FUNCTION "FC_GRP_83" : VOID
TITLE =GROUP =83
{ S7_language := '9(1) Angielski (Stany Zjednoczone)  11.01.2022  09:45:15' }
VERSION : 0.1


VAR_TEMP
  CL : "UDT_CABINET";	//CABINET LOCAL
  CR : "UDT_CABINET";	//CABINET REMOTE
  RelError : BOOL ;	//ERROR RELEASE
  RelErrorCL : BOOL ;	//ERROR RELEASE FROM CABINET LOCAL
  RelErrorCR : BOOL ;	//ERROR RELEASE FROM CABINET REMOTE
  RelControl : BOOL ;	//CONTROL RELEASE
  RelControlCL : BOOL ;	//CONTROL RELEASE FROM CABINET LOCAL
  RelControlCR : BOOL ;	//CONTROL RELEASE FROM CABINET REMOTE
  ErrorConfirm : BOOL ;	//ERROR CONFIRM
  AutoOn : BOOL ;	//AUTOMATIC ON
  AutoOff : BOOL ;	//AUTOMATIC OFF
  LAMP_ON : BOOL ;
END_VAR
BEGIN
NETWORK
TITLE =GLOBAL SIGNALS
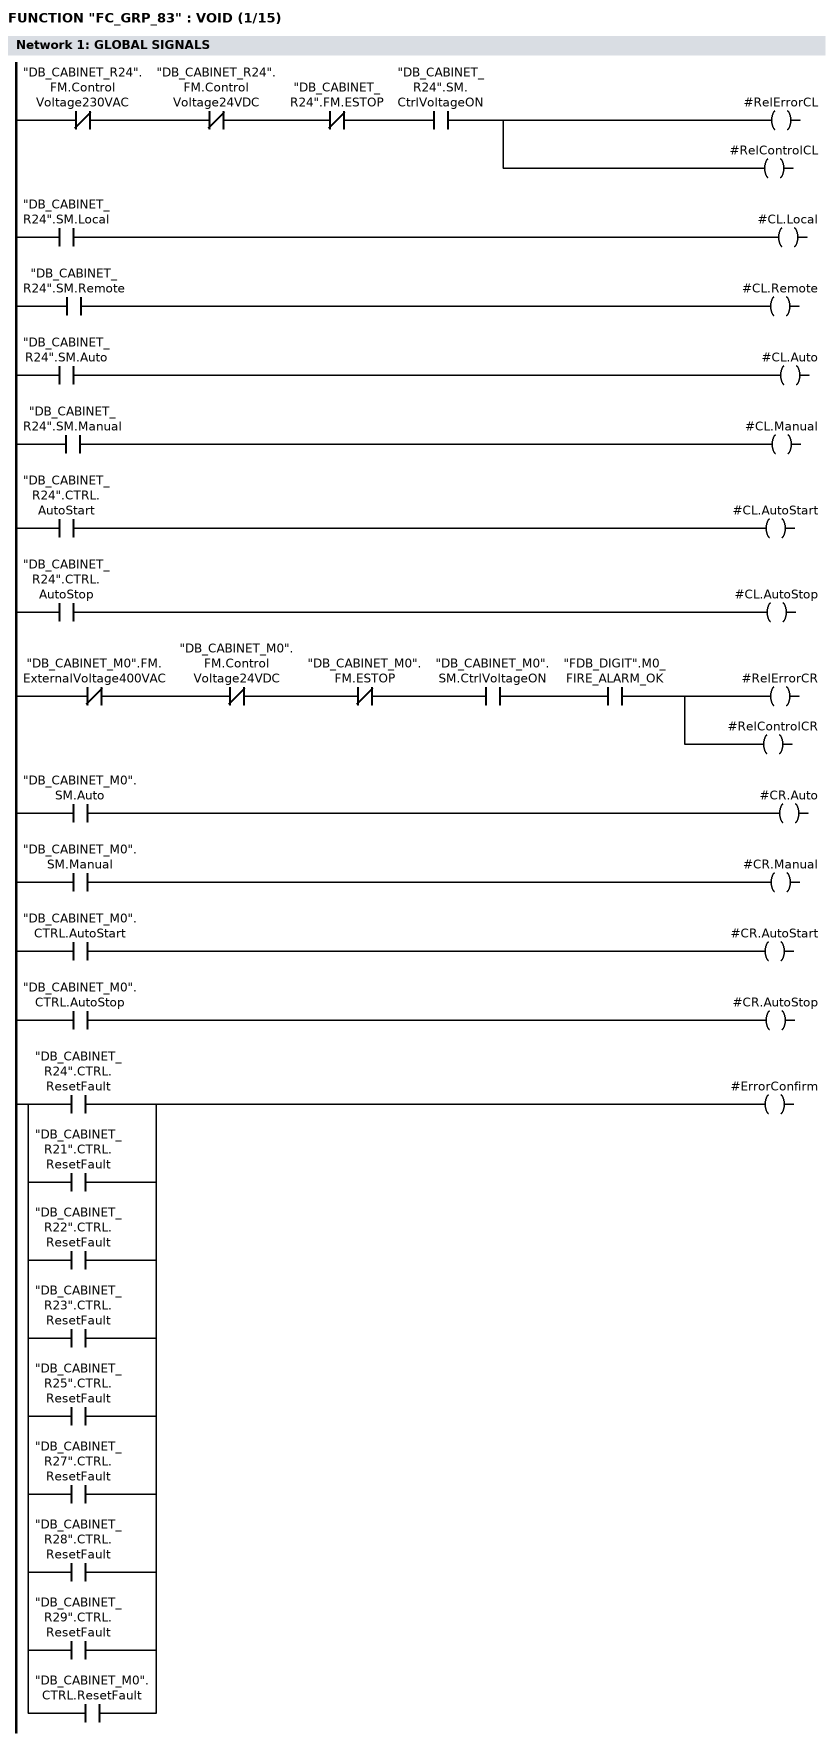
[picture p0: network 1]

// LOCAL
      UN    "DB_CABINET_R24".FM.ControlVoltage230VAC;
      UN    "DB_CABINET_R24".FM.ControlVoltage24VDC;
//      UN    "DB_CABINET_R24".FM.ControlVoltage230VAC_MS
      UN    "DB_CABINET_R24".FM.ESTOP;
      U     "DB_CABINET_R24".SM.CtrlVoltageON;
      =     #RelErrorCL;
      =     #RelControlCL;

      U     "DB_CABINET_R24".SM.Local;
      =     #CL.Local;
      U     "DB_CABINET_R24".SM.Remote;
      =     #CL.Remote;
      U     "DB_CABINET_R24".SM.Auto;
      =     #CL.Auto;
      U     "DB_CABINET_R24".SM.Manual;
      =     #CL.Manual;
      U     "DB_CABINET_R24".CTRL.AutoStart;
      =     #CL.AutoStart;
      U     "DB_CABINET_R24".CTRL.AutoStop;
      =     #CL.AutoStop;

// REMOTE
      UN    "DB_CABINET_M0".FM.ExternalVoltage400VAC;
      UN    "DB_CABINET_M0".FM.ControlVoltage24VDC;
//      UN    "DB_CABINET_M0".FM.ControlVoltage230VAC_MS
      UN    "DB_CABINET_M0".FM.ESTOP;
      U     "DB_CABINET_M0".SM.CtrlVoltageON;
      U     "FDB_DIGIT".M0_FIRE_ALARM_OK;
      =     #RelErrorCR;
      =     #RelControlCR;

      U     "DB_CABINET_M0".SM.Auto;
      =     #CR.Auto;
      U     "DB_CABINET_M0".SM.Manual;
      =     #CR.Manual;
      U     "DB_CABINET_M0".CTRL.AutoStart;
      =     #CR.AutoStart;
      U     "DB_CABINET_M0".CTRL.AutoStop;
      =     #CR.AutoStop;


      U     "DB_CABINET_R24".CTRL.ResetFault;
      O     "DB_CABINET_R21".CTRL.ResetFault;
      O     "DB_CABINET_R22".CTRL.ResetFault;
      O     "DB_CABINET_R23".CTRL.ResetFault;
      O     "DB_CABINET_R25".CTRL.ResetFault;
      O     "DB_CABINET_R27".CTRL.ResetFault;
      O     "DB_CABINET_R28".CTRL.ResetFault;
      O     "DB_CABINET_R29".CTRL.ResetFault;
      O     "DB_CABINET_M0".CTRL.ResetFault;
      =     #ErrorConfirm;

NETWORK
TITLE ==83FTR20-B33 FILTER PRESSURE MONITORING
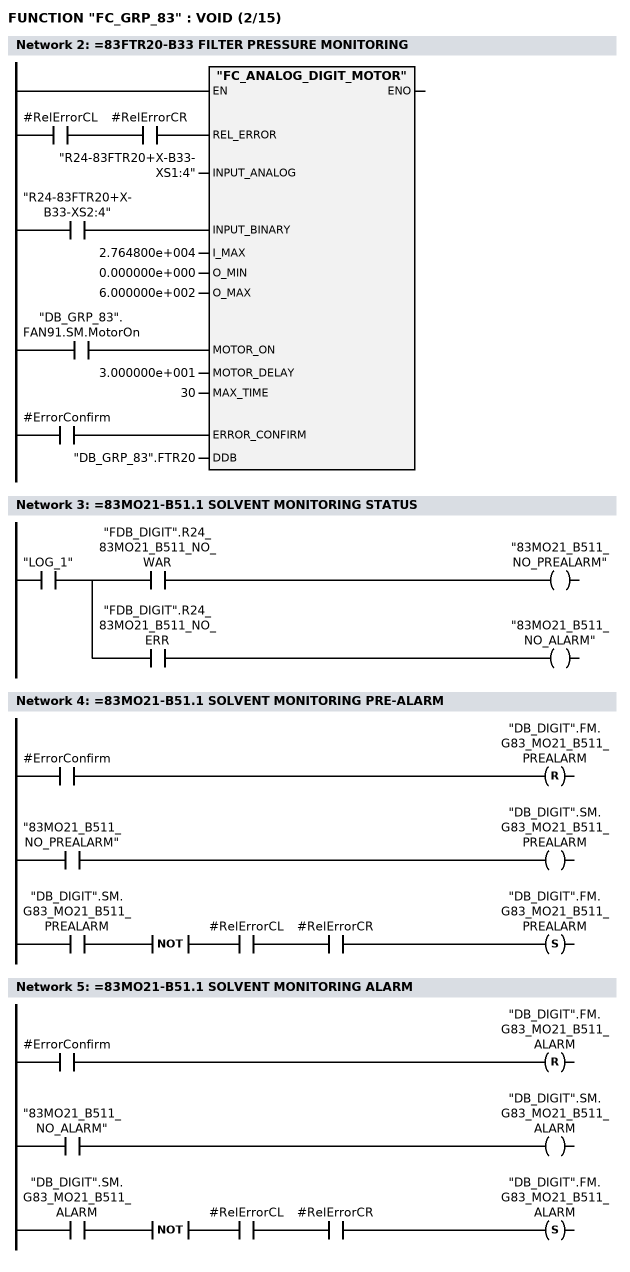
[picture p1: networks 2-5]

      U     #RelErrorCL;
      U     #RelErrorCR;
      =     L      6.0;
      BLD   103;
      U     "R24-83FTR20+X-B33-XS2:4";
      =     L      6.1;
      BLD   103;
      U     "DB_GRP_83".FAN91.SM.MotorOn;
      =     L      6.2;
      BLD   103;
      U     #ErrorConfirm;
      =     L      6.3;
      BLD   103;
      CALL "FC_ANALOG_DIGIT_MOTOR" (
           REL_ERROR                := L      6.0,
           INPUT_ANALOG             := "R24-83FTR20+X-B33-XS1:4",
           INPUT_BINARY             := L      6.1,
           I_MAX                    := 2.764800e+004,
           O_MIN                    := 0.000000e+000,
           O_MAX                    := 6.000000e+002,
           MOTOR_ON                 := L      6.2,
           MOTOR_DELAY              := 3.000000e+001,
           MAX_TIME                 := 30,
           ERROR_CONFIRM            := L      6.3,
           DDB                      := "DB_GRP_83".FTR20);
      NOP   0;
NETWORK
TITLE ==83MO21-B51.1 SOLVENT MONITORING STATUS

      U     "LOG_1";
      =     L      6.0;
      U     L      6.0;
      U     "FDB_DIGIT".R24_83MO21_B511_NO_WAR;
      =     "83MO21_B511_NO_PREALARM";
      U     L      6.0;
      U     "FDB_DIGIT".R24_83MO21_B511_NO_ERR;
      =     "83MO21_B511_NO_ALARM";
NETWORK
TITLE ==83MO21-B51.1 SOLVENT MONITORING PRE-ALARM

      U     #ErrorConfirm;
      R     "DB_DIGIT".FM.G83_MO21_B511_PREALARM;
      U     "83MO21_B511_NO_PREALARM";
      =     "DB_DIGIT".SM.G83_MO21_B511_PREALARM;
      U     "DB_DIGIT".SM.G83_MO21_B511_PREALARM;
      NOT   ;
      U     #RelErrorCL;
      U     #RelErrorCR;
      S     "DB_DIGIT".FM.G83_MO21_B511_PREALARM;
      NOP   0;
NETWORK
TITLE ==83MO21-B51.1 SOLVENT MONITORING ALARM

      U     #ErrorConfirm;
      R     "DB_DIGIT".FM.G83_MO21_B511_ALARM;
      U     "83MO21_B511_NO_ALARM";
      =     "DB_DIGIT".SM.G83_MO21_B511_ALARM;
      U     "DB_DIGIT".SM.G83_MO21_B511_ALARM;
      NOT   ;
      U     #RelErrorCL;
      U     #RelErrorCR;
      S     "DB_DIGIT".FM.G83_MO21_B511_ALARM;
      NOP   0;
NETWORK
TITLE ==83MO21-B51.1 SOLVENT MONITORING ANALOG
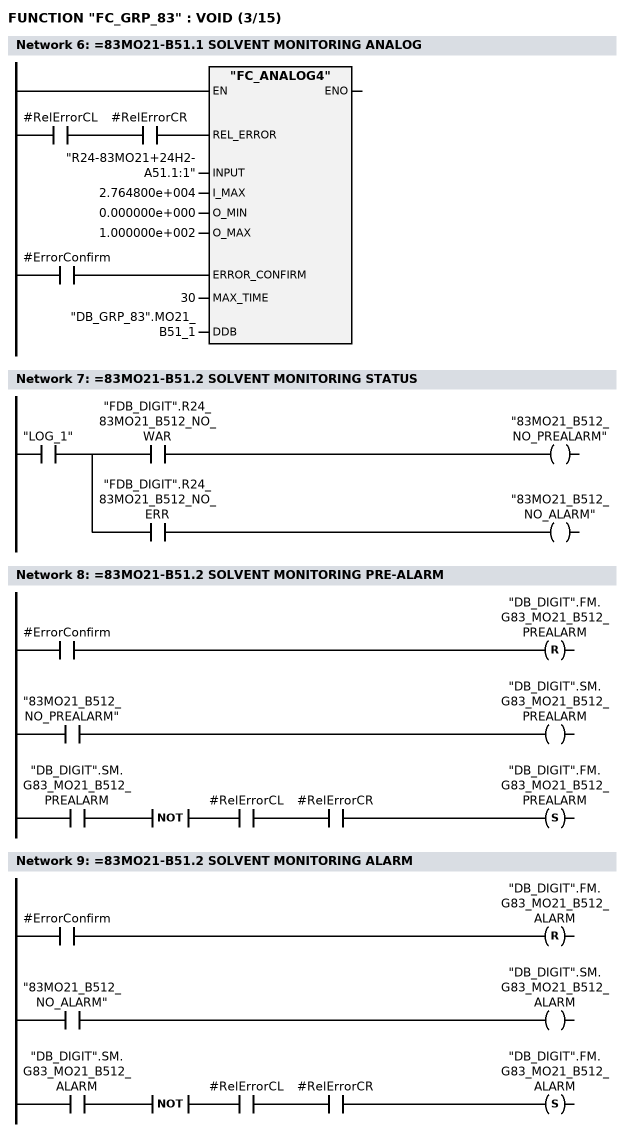
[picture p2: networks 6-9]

      U     #RelErrorCL;
      U     #RelErrorCR;
      =     L      6.0;
      BLD   103;
      U     #ErrorConfirm;
      =     L      6.1;
      BLD   103;
      CALL "FC_ANALOG4" (
           REL_ERROR                := L      6.0,
           INPUT                    := "R24-83MO21+24H2-A51.1:1",
           I_MAX                    := 2.764800e+004,
           O_MIN                    := 0.000000e+000,
           O_MAX                    := 1.000000e+002,
           ERROR_CONFIRM            := L      6.1,
           MAX_TIME                 := 30,
           DDB                      := "DB_GRP_83".MO21_B51_1);
      NOP   0;
NETWORK
TITLE ==83MO21-B51.2 SOLVENT MONITORING STATUS

      U     "LOG_1";
      =     L      6.0;
      U     L      6.0;
      U     "FDB_DIGIT".R24_83MO21_B512_NO_WAR;
      =     "83MO21_B512_NO_PREALARM";
      U     L      6.0;
      U     "FDB_DIGIT".R24_83MO21_B512_NO_ERR;
      =     "83MO21_B512_NO_ALARM";
NETWORK
TITLE ==83MO21-B51.2 SOLVENT MONITORING PRE-ALARM

      U     #ErrorConfirm;
      R     "DB_DIGIT".FM.G83_MO21_B512_PREALARM;
      U     "83MO21_B512_NO_PREALARM";
      =     "DB_DIGIT".SM.G83_MO21_B512_PREALARM;
      U     "DB_DIGIT".SM.G83_MO21_B512_PREALARM;
      NOT   ;
      U     #RelErrorCL;
      U     #RelErrorCR;
      S     "DB_DIGIT".FM.G83_MO21_B512_PREALARM;
      NOP   0;
NETWORK
TITLE ==83MO21-B51.2 SOLVENT MONITORING ALARM

      U     #ErrorConfirm;
      R     "DB_DIGIT".FM.G83_MO21_B512_ALARM;
      U     "83MO21_B512_NO_ALARM";
      =     "DB_DIGIT".SM.G83_MO21_B512_ALARM;
      U     "DB_DIGIT".SM.G83_MO21_B512_ALARM;
      NOT   ;
      U     #RelErrorCL;
      U     #RelErrorCR;
      S     "DB_DIGIT".FM.G83_MO21_B512_ALARM;
      NOP   0;
NETWORK
TITLE ==83MO21-B51.2 SOLVENT MONITORING ANALOG
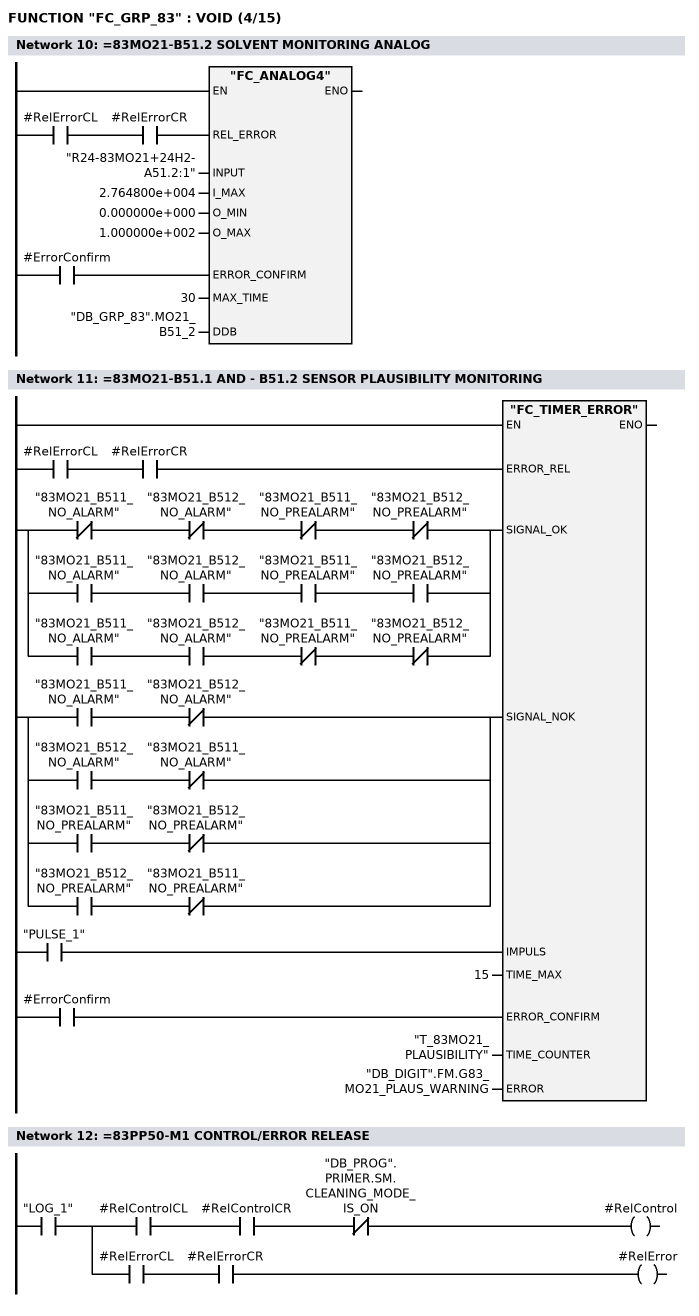
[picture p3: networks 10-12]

      U     #RelErrorCL;
      U     #RelErrorCR;
      =     L      6.0;
      BLD   103;
      U     #ErrorConfirm;
      =     L      6.1;
      BLD   103;
      CALL "FC_ANALOG4" (
           REL_ERROR                := L      6.0,
           INPUT                    := "R24-83MO21+24H2-A51.2:1",
           I_MAX                    := 2.764800e+004,
           O_MIN                    := 0.000000e+000,
           O_MAX                    := 1.000000e+002,
           ERROR_CONFIRM            := L      6.1,
           MAX_TIME                 := 30,
           DDB                      := "DB_GRP_83".MO21_B51_2);
      NOP   0;
NETWORK
TITLE ==83MO21-B51.1 AND - B51.2 SENSOR PLAUSIBILITY MONITORING

      U     #RelErrorCL;
      U     #RelErrorCR;
      =     L      6.0;
      BLD   103;
      U(    ;
      UN    "83MO21_B511_NO_ALARM";
      UN    "83MO21_B512_NO_ALARM";
      UN    "83MO21_B511_NO_PREALARM";
      UN    "83MO21_B512_NO_PREALARM";
      O     ;
      U     "83MO21_B511_NO_ALARM";
      U     "83MO21_B512_NO_ALARM";
      U     "83MO21_B511_NO_PREALARM";
      U     "83MO21_B512_NO_PREALARM";
      O     ;
      U     "83MO21_B511_NO_ALARM";
      U     "83MO21_B512_NO_ALARM";
      UN    "83MO21_B511_NO_PREALARM";
      UN    "83MO21_B512_NO_PREALARM";
      )     ;
      =     L      6.1;
      BLD   103;
      U(    ;
      U     "83MO21_B511_NO_ALARM";
      UN    "83MO21_B512_NO_ALARM";
      O     ;
      U     "83MO21_B512_NO_ALARM";
      UN    "83MO21_B511_NO_ALARM";
      O     ;
      U     "83MO21_B511_NO_PREALARM";
      UN    "83MO21_B512_NO_PREALARM";
      O     ;
      U     "83MO21_B512_NO_PREALARM";
      UN    "83MO21_B511_NO_PREALARM";
      )     ;
      =     L      6.2;
      BLD   103;
      U     "PULSE_1";
      =     L      6.3;
      BLD   103;
      U     #ErrorConfirm;
      =     L      6.4;
      BLD   103;
      CALL "FC_TIMER_ERROR" (
           ERROR_REL                := L      6.0,
           SIGNAL_OK                := L      6.1,
           SIGNAL_NOK               := L      6.2,
           IMPULS                   := L      6.3,
           TIME_MAX                 := 15,
           ERROR_CONFIRM            := L      6.4,
           TIME_COUNTER             := "T_83MO21_PLAUSIBILITY",
           ERROR                    := "DB_DIGIT".FM.G83_MO21_PLAUS_WARNING);
      NOP   0;
NETWORK
TITLE ==83PP50-M1 CONTROL/ERROR RELEASE

      U     "LOG_1";
      =     L      6.0;
      U     L      6.0;
      U     #RelControlCL;
      U     #RelControlCR;
      UN    "DB_PROG".PRIMER.SM.CLEANING_MODE_IS_ON;
      =     #RelControl;
      U     L      6.0;
      U     #RelErrorCL;
      U     #RelErrorCR;
      =     #RelError;
NETWORK
TITLE ==83PP50/51 TEMPERATURE TIMER
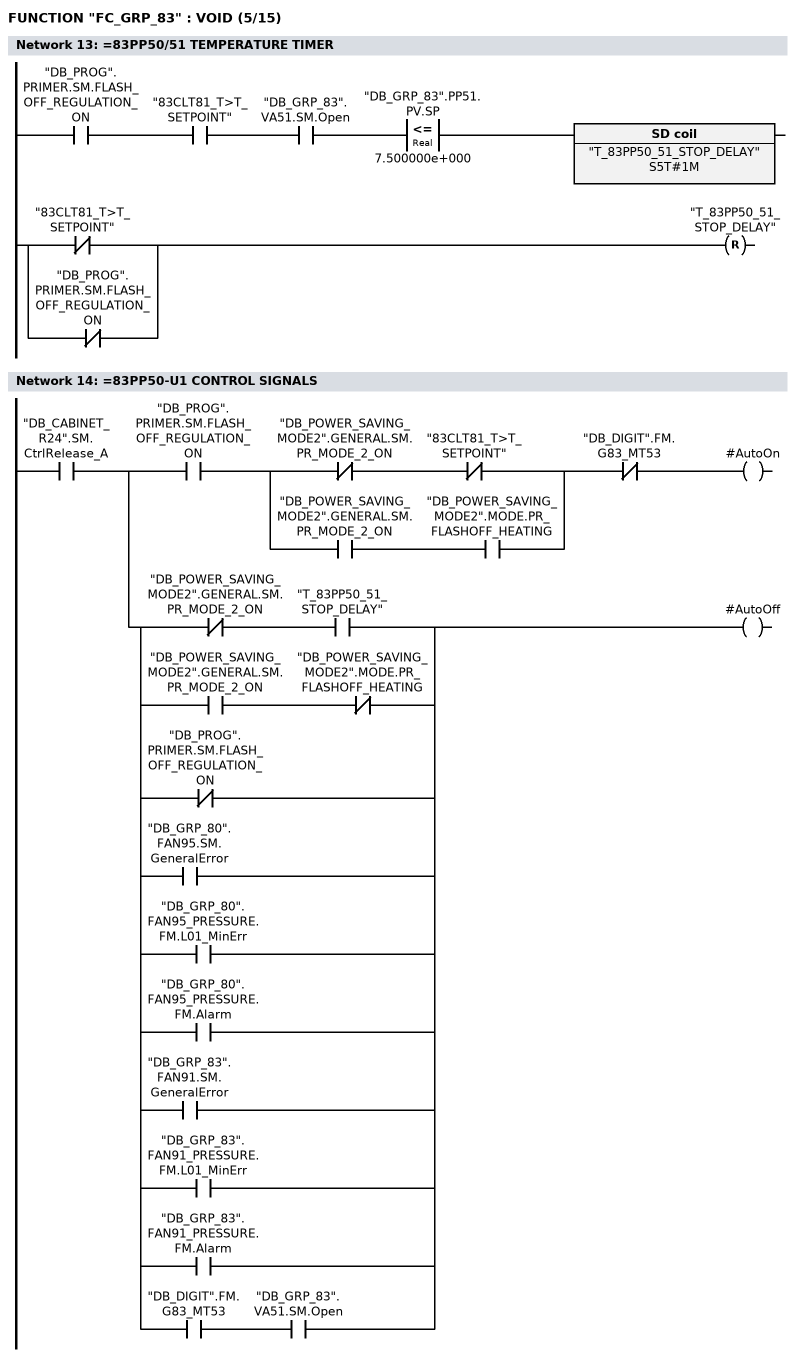
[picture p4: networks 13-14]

      U     "DB_PROG".PRIMER.SM.FLASH_OFF_REGULATION_ON;
      U     "83CLT81_T>T_SETPOINT";
      U     "DB_GRP_83".VA51.SM.Open;
      U(    ;
      L     "DB_GRP_83".PP51.PV.SP;
      L     7.500000e+000;
      <=R   ;
      )     ;
      L     S5T#1M;
      SE    "T_83PP50_51_STOP_DELAY";
      U(    ;
      ON    "83CLT81_T>T_SETPOINT";
      ON    "DB_PROG".PRIMER.SM.FLASH_OFF_REGULATION_ON;
      )     ;
      R     "T_83PP50_51_STOP_DELAY";
      NOP   0;
      NOP   0;
      NOP   0;
NETWORK
TITLE ==83PP50-U1 CONTROL SIGNALS

      U     "DB_CABINET_R24".SM.CtrlRelease_A;
      =     L      6.0;
      U     L      6.0;
      U     "DB_PROG".PRIMER.SM.FLASH_OFF_REGULATION_ON;
      U(    ;
      UN    "DB_POWER_SAVING_MODE2".GENERAL.SM.PR_MODE_2_ON;
      UN    "83CLT81_T>T_SETPOINT";
      O     ;
      U     "DB_POWER_SAVING_MODE2".GENERAL.SM.PR_MODE_2_ON;
      U     "DB_POWER_SAVING_MODE2".MODE.PR_FLASHOFF_HEATING;
      )     ;
      UN    "DB_DIGIT".FM.G83_MT53;
      =     #AutoOn;
      U     L      6.0;
      U(    ;
      UN    "DB_POWER_SAVING_MODE2".GENERAL.SM.PR_MODE_2_ON;
      U     "T_83PP50_51_STOP_DELAY";
      O     ;
      U     "DB_POWER_SAVING_MODE2".GENERAL.SM.PR_MODE_2_ON;
      UN    "DB_POWER_SAVING_MODE2".MODE.PR_FLASHOFF_HEATING;
      ON    "DB_PROG".PRIMER.SM.FLASH_OFF_REGULATION_ON;
      O     "DB_GRP_80".FAN95.SM.GeneralError;
      O     "DB_GRP_80".FAN95_PRESSURE.FM.L01_MinErr;
      O     "DB_GRP_80".FAN95_PRESSURE.FM.Alarm;
      O     "DB_GRP_83".FAN91.SM.GeneralError;
      O     "DB_GRP_83".FAN91_PRESSURE.FM.L01_MinErr;
      O     "DB_GRP_83".FAN91_PRESSURE.FM.Alarm;
      O     ;
      U     "DB_DIGIT".FM.G83_MT53;
      U     "DB_GRP_83".VA51.SM.Open;
      )     ;
      =     #AutoOff;
NETWORK
TITLE ==83PP50-M1 HEATING PUMP
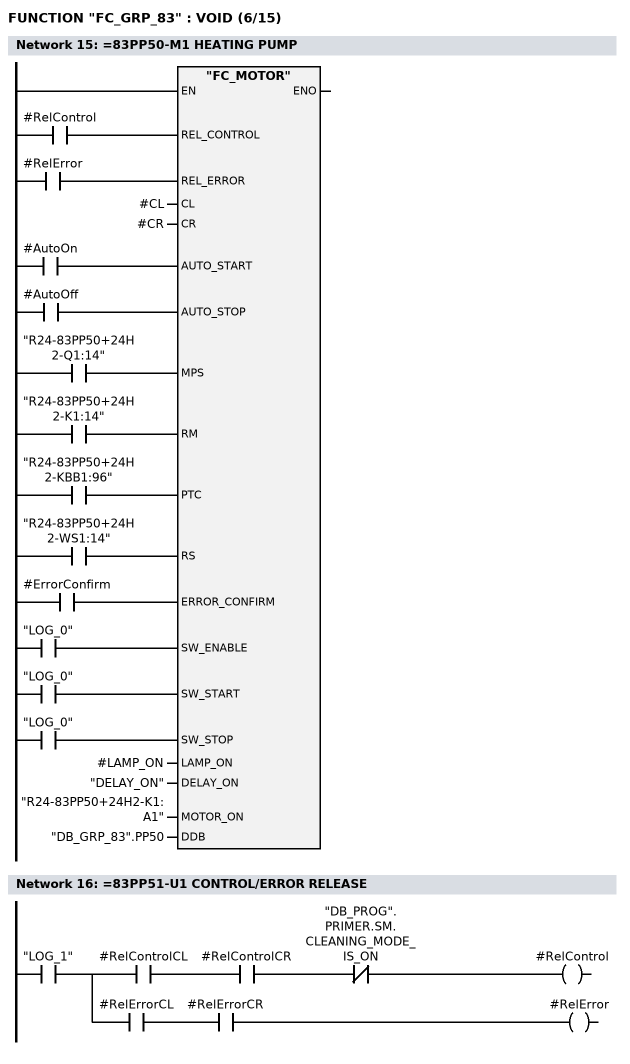
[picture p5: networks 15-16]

      U     #RelControl;
      =     L      6.0;
      BLD   103;
      U     #RelError;
      =     L      6.1;
      BLD   103;
      U     #AutoOn;
      =     L      6.2;
      BLD   103;
      U     #AutoOff;
      =     L      6.3;
      BLD   103;
      U     "R24-83PP50+24H2-Q1:14";
      =     L      6.4;
      BLD   103;
      U     "R24-83PP50+24H2-K1:14";
      =     L      6.5;
      BLD   103;
      U     "R24-83PP50+24H2-KBB1:96";
      =     L      6.6;
      BLD   103;
      U     "R24-83PP50+24H2-WS1:14";
      =     L      6.7;
      BLD   103;
      U     #ErrorConfirm;
      =     L      7.0;
      BLD   103;
      U     "LOG_0";
      =     L      7.1;
      BLD   103;
      U     "LOG_0";
      =     L      7.2;
      BLD   103;
      U     "LOG_0";
      =     L      7.3;
      BLD   103;
      CALL "FC_MOTOR" (
           REL_CONTROL              := L      6.0,
           REL_ERROR                := L      6.1,
           CL                       := #CL,
           CR                       := #CR,
           AUTO_START               := L      6.2,
           AUTO_STOP                := L      6.3,
           MPS                      := L      6.4,
           RM                       := L      6.5,
           PTC                      := L      6.6,
           RS                       := L      6.7,
           ERROR_CONFIRM            := L      7.0,
           SW_ENABLE                := L      7.1,
           SW_START                 := L      7.2,
           SW_STOP                  := L      7.3,
           LAMP_ON                  := #LAMP_ON,
           DELAY_ON                 := "DELAY_ON",
           MOTOR_ON                 := "R24-83PP50+24H2-K1:A1",
           DDB                      := "DB_GRP_83".PP50);
      NOP   0;
NETWORK
TITLE ==83PP51-U1 CONTROL/ERROR RELEASE

      U     "LOG_1";
      =     L      6.0;
      U     L      6.0;
      U     #RelControlCL;
      U     #RelControlCR;
      UN    "DB_PROG".PRIMER.SM.CLEANING_MODE_IS_ON;
      =     #RelControl;
      U     L      6.0;
      U     #RelErrorCL;
      U     #RelErrorCR;
      =     #RelError;
NETWORK
TITLE ==83PP51-U1 CONTROL SIGNALS
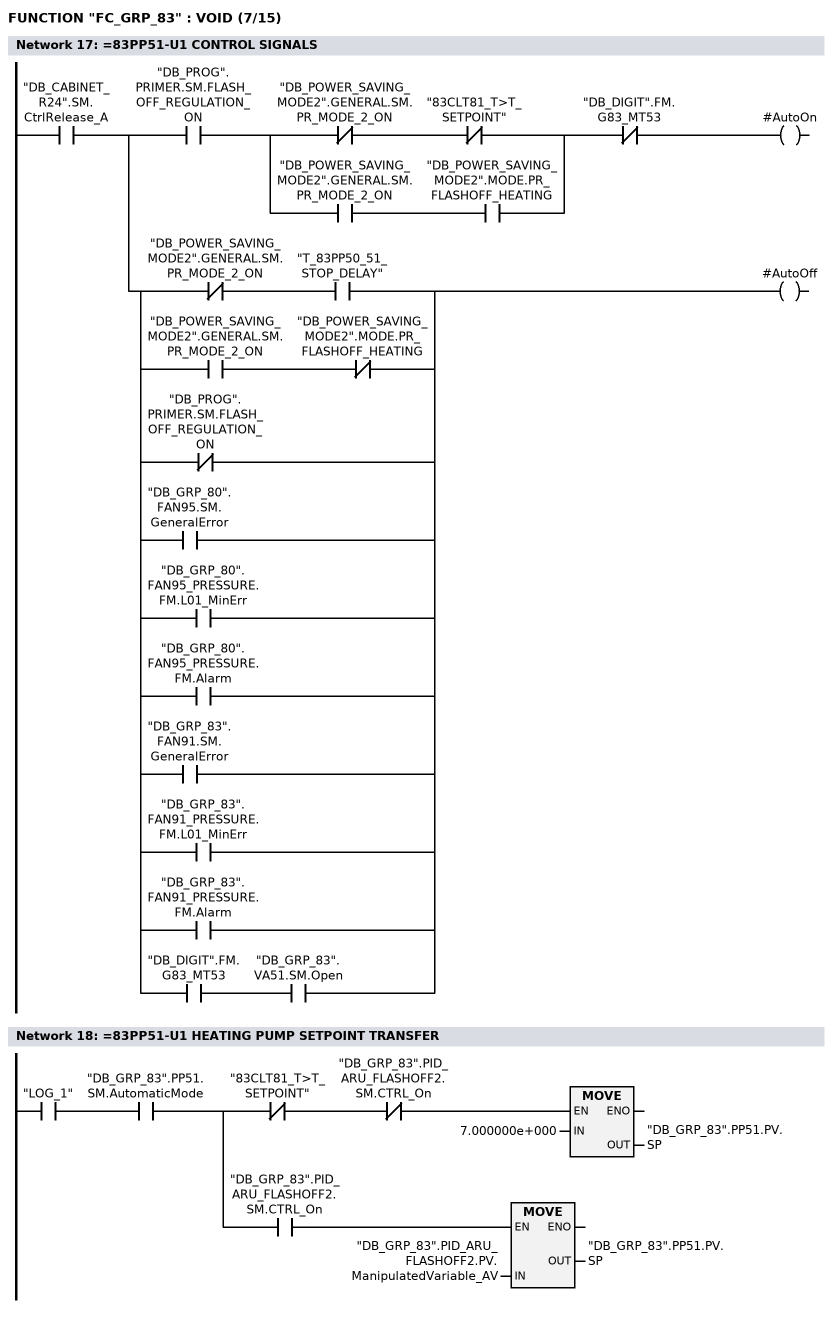
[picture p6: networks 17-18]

      U     "DB_CABINET_R24".SM.CtrlRelease_A;
      =     L      6.0;
      U     L      6.0;
      U     "DB_PROG".PRIMER.SM.FLASH_OFF_REGULATION_ON;
      U(    ;
      UN    "DB_POWER_SAVING_MODE2".GENERAL.SM.PR_MODE_2_ON;
      UN    "83CLT81_T>T_SETPOINT";
      O     ;
      U     "DB_POWER_SAVING_MODE2".GENERAL.SM.PR_MODE_2_ON;
      U     "DB_POWER_SAVING_MODE2".MODE.PR_FLASHOFF_HEATING;
      )     ;
      UN    "DB_DIGIT".FM.G83_MT53;
      =     #AutoOn;
      U     L      6.0;
      U(    ;
      UN    "DB_POWER_SAVING_MODE2".GENERAL.SM.PR_MODE_2_ON;
      U     "T_83PP50_51_STOP_DELAY";
      O     ;
      U     "DB_POWER_SAVING_MODE2".GENERAL.SM.PR_MODE_2_ON;
      UN    "DB_POWER_SAVING_MODE2".MODE.PR_FLASHOFF_HEATING;
      ON    "DB_PROG".PRIMER.SM.FLASH_OFF_REGULATION_ON;
      O     "DB_GRP_80".FAN95.SM.GeneralError;
      O     "DB_GRP_80".FAN95_PRESSURE.FM.L01_MinErr;
      O     "DB_GRP_80".FAN95_PRESSURE.FM.Alarm;
      O     "DB_GRP_83".FAN91.SM.GeneralError;
      O     "DB_GRP_83".FAN91_PRESSURE.FM.L01_MinErr;
      O     "DB_GRP_83".FAN91_PRESSURE.FM.Alarm;
      O     ;
      U     "DB_DIGIT".FM.G83_MT53;
      U     "DB_GRP_83".VA51.SM.Open;
      )     ;
      =     #AutoOff;
NETWORK
TITLE ==83PP51-U1 HEATING PUMP SETPOINT TRANSFER

      U     "LOG_1";
      U     "DB_GRP_83".PP51.SM.AutomaticMode;
      =     L      6.0;
      U     L      6.0;
      UN    "83CLT81_T>T_SETPOINT";
      UN    "DB_GRP_83".PID_ARU_FLASHOFF2.SM.CTRL_On;
      SPBNB _001;
      L     7.000000e+000;
      T     "DB_GRP_83".PP51.PV.SP;
_001: NOP   0;
      U     L      6.0;
      U     "DB_GRP_83".PID_ARU_FLASHOFF2.SM.CTRL_On;
      SPBNB _002;
      L     "DB_GRP_83".PID_ARU_FLASHOFF2.PV.ManipulatedVariable_AV;
      T     "DB_GRP_83".PP51.PV.SP;
_002: NOP   0;
NETWORK
TITLE ==83PP51-U1 HEATING PUMP
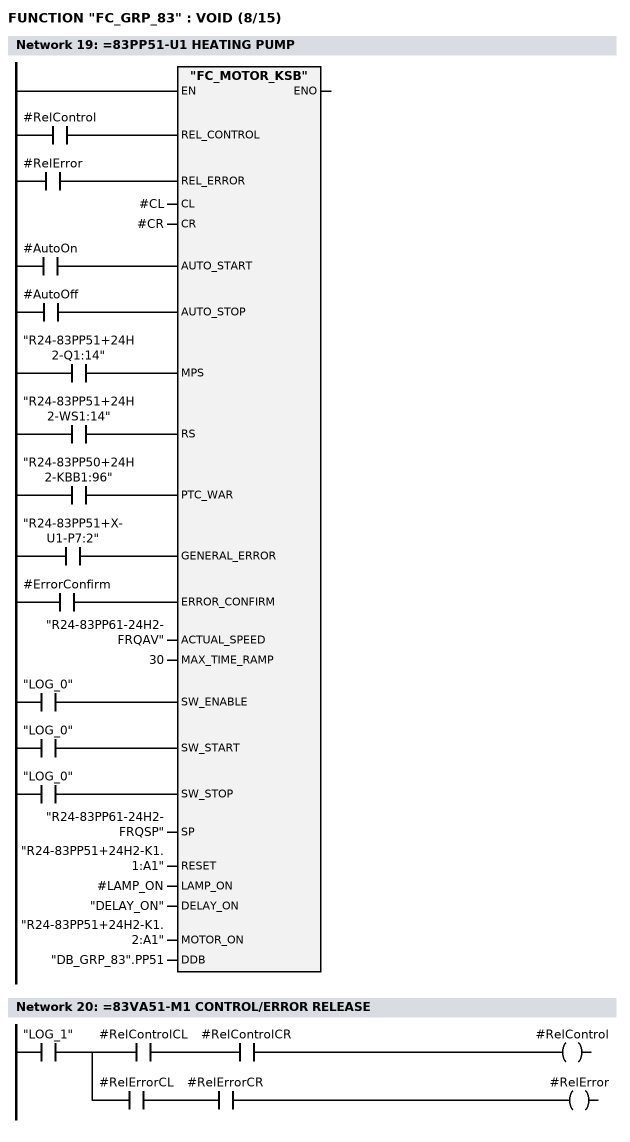
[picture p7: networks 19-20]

      U     #RelControl;
      =     L      6.0;
      BLD   103;
      U     #RelError;
      =     L      6.1;
      BLD   103;
      U     #AutoOn;
      =     L      6.2;
      BLD   103;
      U     #AutoOff;
      =     L      6.3;
      BLD   103;
      U     "R24-83PP51+24H2-Q1:14";
      =     L      6.4;
      BLD   103;
      U     "R24-83PP51+24H2-WS1:14";
      =     L      6.5;
      BLD   103;
      U     "R24-83PP50+24H2-KBB1:96";
      =     L      6.6;
      BLD   103;
      U     "R24-83PP51+X-U1-P7:2";
      =     L      6.7;
      BLD   103;
      U     #ErrorConfirm;
      =     L      7.0;
      BLD   103;
      U     "LOG_0";
      =     L      7.1;
      BLD   103;
      U     "LOG_0";
      =     L      7.2;
      BLD   103;
      U     "LOG_0";
      =     L      7.3;
      BLD   103;
      CALL "FC_MOTOR_KSB" (
           REL_CONTROL              := L      6.0,
           REL_ERROR                := L      6.1,
           CL                       := #CL,
           CR                       := #CR,
           AUTO_START               := L      6.2,
           AUTO_STOP                := L      6.3,
           MPS                      := L      6.4,
           RS                       := L      6.5,
           PTC_WAR                  := L      6.6,
           GENERAL_ERROR            := L      6.7,
           ERROR_CONFIRM            := L      7.0,
           ACTUAL_SPEED             := "R24-83PP61-24H2-FRQAV",
           MAX_TIME_RAMP            := 30,
           SW_ENABLE                := L      7.1,
           SW_START                 := L      7.2,
           SW_STOP                  := L      7.3,
           SP                       := "R24-83PP61-24H2-FRQSP",
           RESET                    := "R24-83PP51+24H2-K1.1:A1",
           LAMP_ON                  := #LAMP_ON,
           DELAY_ON                 := "DELAY_ON",
           MOTOR_ON                 := "R24-83PP51+24H2-K1.2:A1",
           DDB                      := "DB_GRP_83".PP51);
      NOP   0;
NETWORK
TITLE ==83VA51-M1 CONTROL/ERROR RELEASE

      U     "LOG_1";
      =     L      6.0;
      U     L      6.0;
      U     #RelControlCL;
      U     #RelControlCR;
      =     #RelControl;
      U     L      6.0;
      U     #RelErrorCL;
      U     #RelErrorCR;
      =     #RelError;
NETWORK
TITLE ==83VA51-M1 HEATING VALVE CONTROL SIGNALS
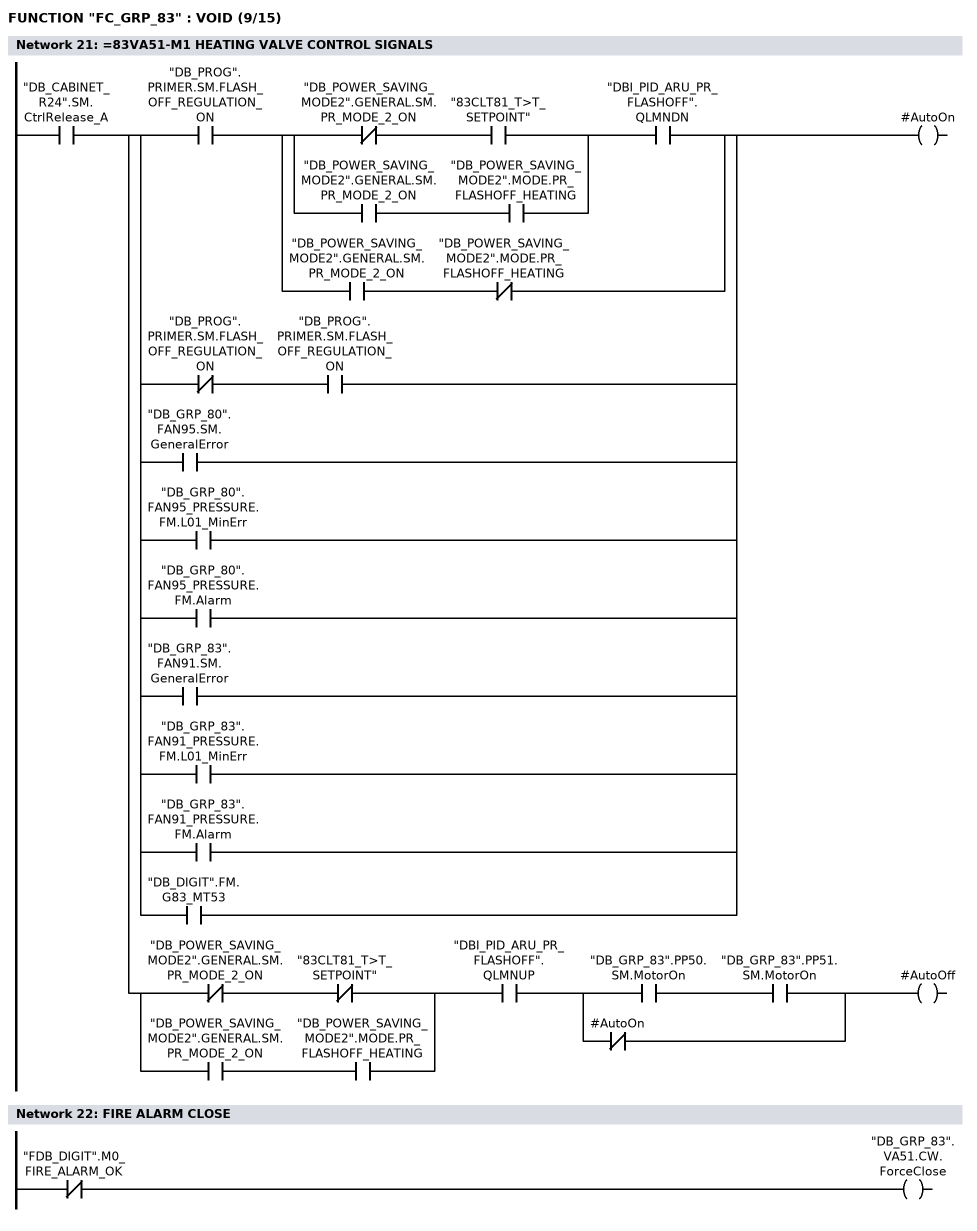
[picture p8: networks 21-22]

      U     "DB_CABINET_R24".SM.CtrlRelease_A;
      =     L      6.0;
      U     L      6.0;
      U(    ;
      U     "DB_PROG".PRIMER.SM.FLASH_OFF_REGULATION_ON;
      U(    ;
      U(    ;
      UN    "DB_POWER_SAVING_MODE2".GENERAL.SM.PR_MODE_2_ON;
      U     "83CLT81_T>T_SETPOINT";
      O     ;
      U     "DB_POWER_SAVING_MODE2".GENERAL.SM.PR_MODE_2_ON;
      U     "DB_POWER_SAVING_MODE2".MODE.PR_FLASHOFF_HEATING;
      )     ;
      U     "DBI_PID_ARU_PR_FLASHOFF".QLMNDN;
      O     ;
      U     "DB_POWER_SAVING_MODE2".GENERAL.SM.PR_MODE_2_ON;
      UN    "DB_POWER_SAVING_MODE2".MODE.PR_FLASHOFF_HEATING;
      )     ;
      O     ;
      UN    "DB_PROG".PRIMER.SM.FLASH_OFF_REGULATION_ON;
      U     "DB_PROG".PRIMER.SM.FLASH_OFF_REGULATION_ON;
      O     "DB_GRP_80".FAN95.SM.GeneralError;
      O     "DB_GRP_80".FAN95_PRESSURE.FM.L01_MinErr;
      O     "DB_GRP_80".FAN95_PRESSURE.FM.Alarm;
      O     "DB_GRP_83".FAN91.SM.GeneralError;
      O     "DB_GRP_83".FAN91_PRESSURE.FM.L01_MinErr;
      O     "DB_GRP_83".FAN91_PRESSURE.FM.Alarm;
      O     "DB_DIGIT".FM.G83_MT53;
      )     ;
      =     #AutoOn;
      U     L      6.0;
      U(    ;
      UN    "DB_POWER_SAVING_MODE2".GENERAL.SM.PR_MODE_2_ON;
      UN    "83CLT81_T>T_SETPOINT";
      O     ;
      U     "DB_POWER_SAVING_MODE2".GENERAL.SM.PR_MODE_2_ON;
      U     "DB_POWER_SAVING_MODE2".MODE.PR_FLASHOFF_HEATING;
      )     ;
      U     "DBI_PID_ARU_PR_FLASHOFF".QLMNUP;
      U(    ;
      U     "DB_GRP_83".PP50.SM.MotorOn;
      U     "DB_GRP_83".PP51.SM.MotorOn;
      ON    #AutoOn;
      )     ;
      =     #AutoOff;
NETWORK
TITLE =FIRE ALARM CLOSE

      UN    "FDB_DIGIT".M0_FIRE_ALARM_OK;
      =     "DB_GRP_83".VA51.CW.ForceClose;
NETWORK
TITLE ==83VA51-M1 HEATING VALVE CONTROL
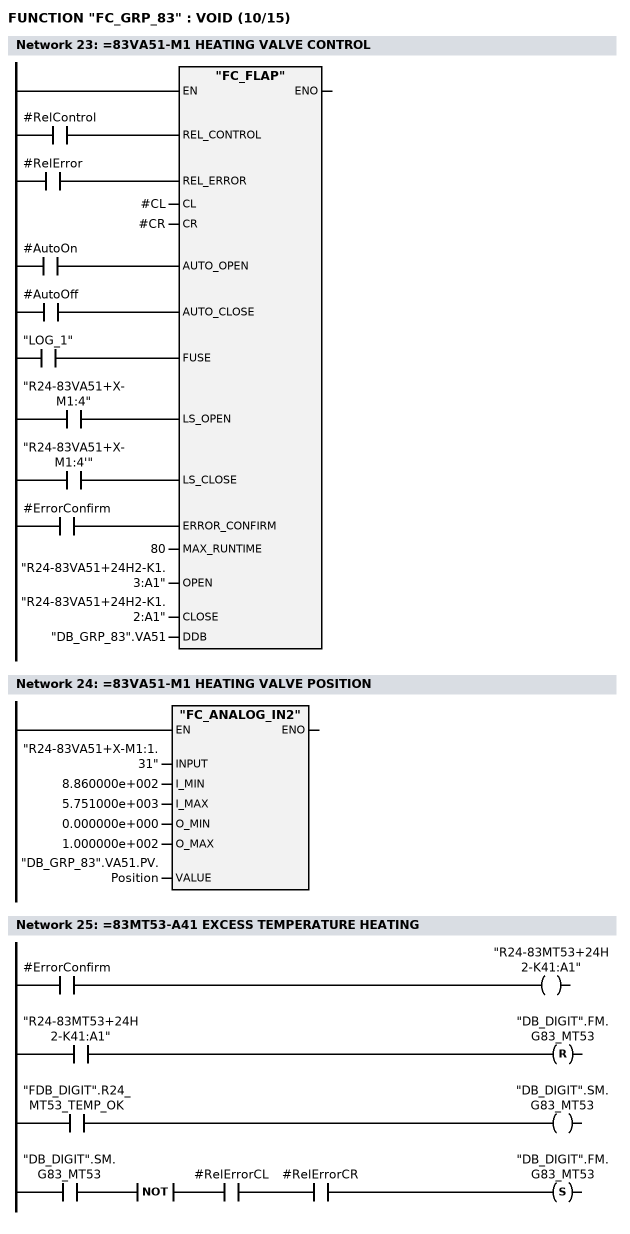
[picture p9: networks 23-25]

      U     #RelControl;
      =     L      6.0;
      BLD   103;
      U     #RelError;
      =     L      6.1;
      BLD   103;
      U     #AutoOn;
      =     L      6.2;
      BLD   103;
      U     #AutoOff;
      =     L      6.3;
      BLD   103;
      U     "LOG_1";
      =     L      6.4;
      BLD   103;
      U     "R24-83VA51+X-M1:4";
      =     L      6.5;
      BLD   103;
      U     "R24-83VA51+X-M1:4'";
      =     L      6.6;
      BLD   103;
      U     #ErrorConfirm;
      =     L      6.7;
      BLD   103;
      CALL "FC_FLAP" (
           REL_CONTROL              := L      6.0,
           REL_ERROR                := L      6.1,
           CL                       := #CL,
           CR                       := #CR,
           AUTO_OPEN                := L      6.2,
           AUTO_CLOSE               := L      6.3,
           FUSE                     := L      6.4,
           LS_OPEN                  := L      6.5,
           LS_CLOSE                 := L      6.6,
           ERROR_CONFIRM            := L      6.7,
           MAX_RUNTIME              := 80,
           OPEN                     := "R24-83VA51+24H2-K1.3:A1",
           CLOSE                    := "R24-83VA51+24H2-K1.2:A1",
           DDB                      := "DB_GRP_83".VA51);
      NOP   0;
NETWORK
TITLE ==83VA51-M1 HEATING VALVE POSITION

      CALL "FC_ANALOG_IN2" (
           INPUT                    := "R24-83VA51+X-M1:1.31",
           I_MIN                    := 8.860000e+002,
           I_MAX                    := 5.751000e+003,
           O_MIN                    := 0.000000e+000,
           O_MAX                    := 1.000000e+002,
           VALUE                    := "DB_GRP_83".VA51.PV.Position);
      NOP   0;
NETWORK
TITLE ==83MT53-A41 EXCESS TEMPERATURE HEATING

      U     #ErrorConfirm;
      =     "R24-83MT53+24H2-K41:A1";
      U     "R24-83MT53+24H2-K41:A1";
      R     "DB_DIGIT".FM.G83_MT53;
      U     "FDB_DIGIT".R24_MT53_TEMP_OK;
      =     "DB_DIGIT".SM.G83_MT53;
      U     "DB_DIGIT".SM.G83_MT53;
      NOT   ;
      U     #RelErrorCL;
      U     #RelErrorCR;
      S     "DB_DIGIT".FM.G83_MT53;
      NOP   0;
NETWORK
TITLE ==83FTR80-B33 FILTER PRESSURE MONITORING
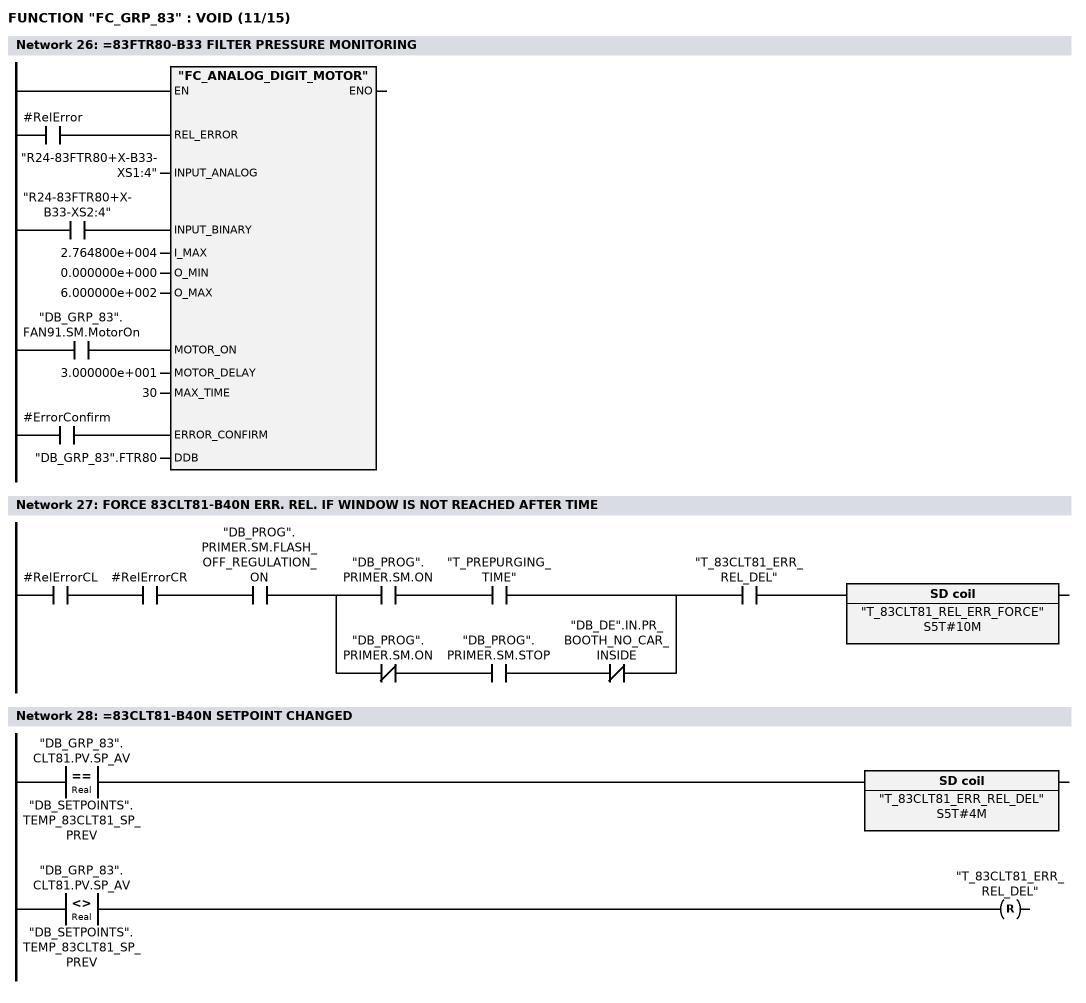
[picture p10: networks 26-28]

      U     #RelError;
      =     L      6.0;
      BLD   103;
      U     "R24-83FTR80+X-B33-XS2:4";
      =     L      6.1;
      BLD   103;
      U     "DB_GRP_83".FAN91.SM.MotorOn;
      =     L      6.2;
      BLD   103;
      U     #ErrorConfirm;
      =     L      6.3;
      BLD   103;
      CALL "FC_ANALOG_DIGIT_MOTOR" (
           REL_ERROR                := L      6.0,
           INPUT_ANALOG             := "R24-83FTR80+X-B33-XS1:4",
           INPUT_BINARY             := L      6.1,
           I_MAX                    := 2.764800e+004,
           O_MIN                    := 0.000000e+000,
           O_MAX                    := 6.000000e+002,
           MOTOR_ON                 := L      6.2,
           MOTOR_DELAY              := 3.000000e+001,
           MAX_TIME                 := 30,
           ERROR_CONFIRM            := L      6.3,
           DDB                      := "DB_GRP_83".FTR80);
      NOP   0;
NETWORK
TITLE =FORCE 83CLT81-B40N ERR. REL. IF WINDOW IS NOT REACHED AFTER TIME

      U     #RelErrorCL;
      U     #RelErrorCR;
      U     "DB_PROG".PRIMER.SM.FLASH_OFF_REGULATION_ON;
      U(    ;
      U     "DB_PROG".PRIMER.SM.ON;
      U     "T_PREPURGING_TIME";
      O     ;
      UN    "DB_PROG".PRIMER.SM.ON;
      U     "DB_PROG".PRIMER.SM.STOP;
      UN    "DB_DE".IN.PR_BOOTH_NO_CAR_INSIDE;
      )     ;
      U     "T_83CLT81_ERR_REL_DEL";
      L     S5T#10M;
      SE    "T_83CLT81_REL_ERR_FORCE";
      NOP   0;
      NOP   0;
      NOP   0;
      NOP   0;
NETWORK
TITLE ==83CLT81-B40N SETPOINT CHANGED

      U(    ;
      L     "DB_GRP_83".CLT81.PV.SP_AV;
      L     "DB_SETPOINTS".TEMP_83CLT81_SP_PREV;
      ==R   ;
      )     ;
      L     S5T#4M;
      SE    "T_83CLT81_ERR_REL_DEL";
      U(    ;
      L     "DB_GRP_83".CLT81.PV.SP_AV;
      L     "DB_SETPOINTS".TEMP_83CLT81_SP_PREV;
      <>R   ;
      )     ;
      R     "T_83CLT81_ERR_REL_DEL";
      NOP   0;
      NOP   0;
      NOP   0;
NETWORK
TITLE ==83CLT81-B40N TEMPERATURE MONITORING
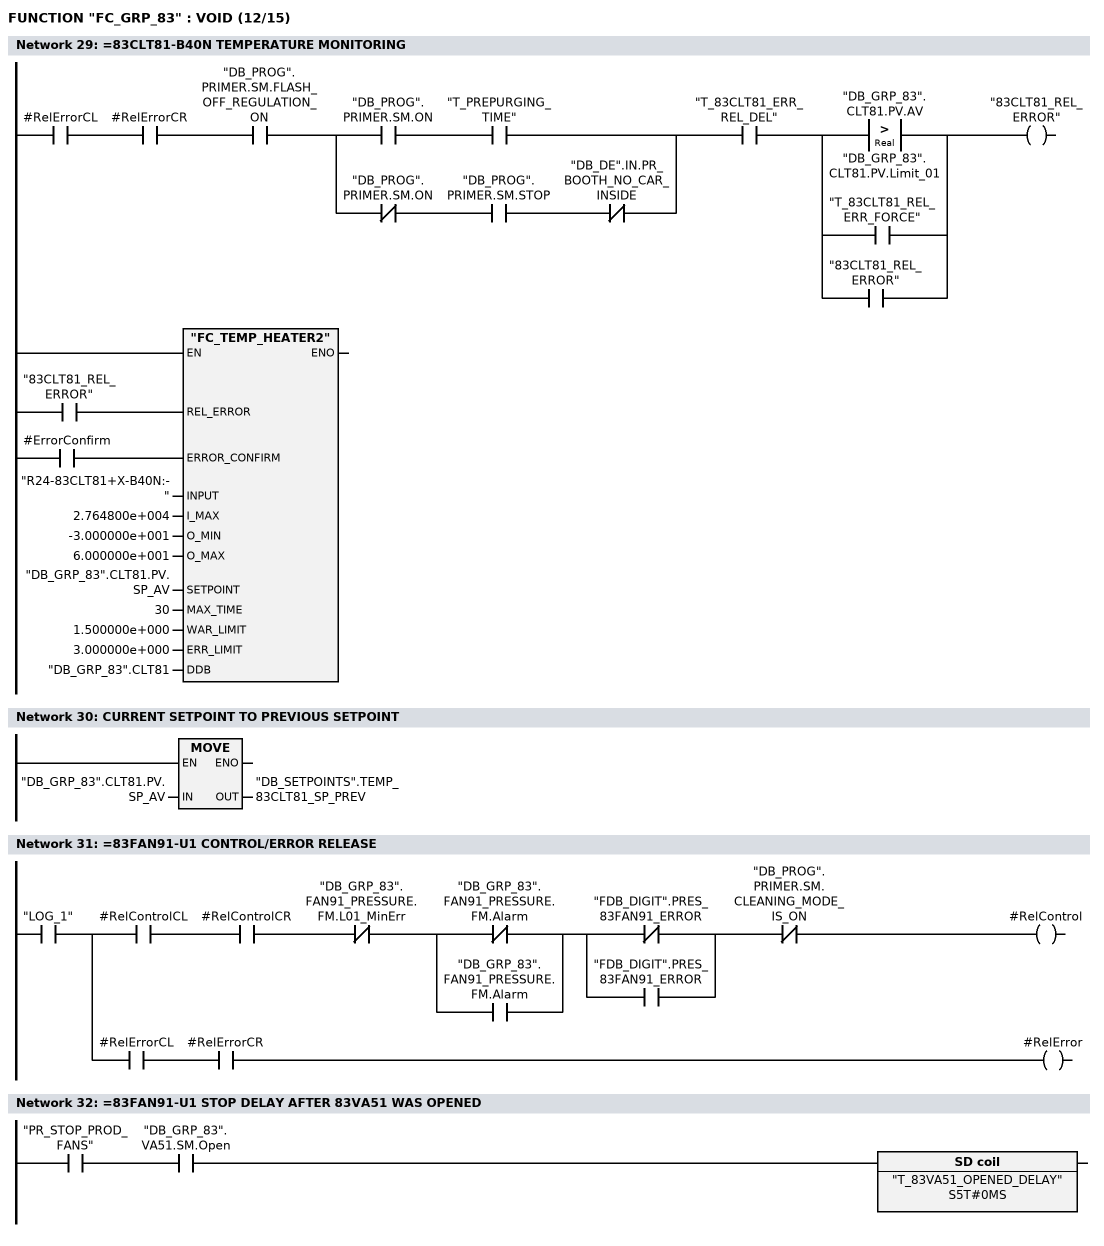
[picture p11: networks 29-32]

      U     #RelErrorCL;
      U     #RelErrorCR;
      U     "DB_PROG".PRIMER.SM.FLASH_OFF_REGULATION_ON;
      U(    ;
      U     "DB_PROG".PRIMER.SM.ON;
      U     "T_PREPURGING_TIME";
      O     ;
      UN    "DB_PROG".PRIMER.SM.ON;
      U     "DB_PROG".PRIMER.SM.STOP;
      UN    "DB_DE".IN.PR_BOOTH_NO_CAR_INSIDE;
      )     ;
      U     "T_83CLT81_ERR_REL_DEL";
      U(    ;
      O(    ;
      L     "DB_GRP_83".CLT81.PV.AV;
      L     "DB_GRP_83".CLT81.PV.Limit_01;
      >R    ;
      )     ;
      O     "T_83CLT81_REL_ERR_FORCE";
      O     "83CLT81_REL_ERROR";
      )     ;
      =     "83CLT81_REL_ERROR";
      U     "83CLT81_REL_ERROR";
      =     L      6.0;
      BLD   103;
      U     #ErrorConfirm;
      =     L      6.1;
      BLD   103;
      CALL "FC_TEMP_HEATER2" (
           REL_ERROR                := L      6.0,
           ERROR_CONFIRM            := L      6.1,
           INPUT                    := "R24-83CLT81+X-B40N:-",
           I_MAX                    := 2.764800e+004,
           O_MIN                    := -3.000000e+001,
           O_MAX                    := 6.000000e+001,
           SETPOINT                 := "DB_GRP_83".CLT81.PV.SP_AV,
           MAX_TIME                 := 30,
           WAR_LIMIT                := 1.500000e+000,
           ERR_LIMIT                := 3.000000e+000,
           DDB                      := "DB_GRP_83".CLT81);
      NOP   0;
NETWORK
TITLE =CURRENT SETPOINT TO PREVIOUS SETPOINT

      L     "DB_GRP_83".CLT81.PV.SP_AV;
      T     "DB_SETPOINTS".TEMP_83CLT81_SP_PREV;
      NOP   0;
NETWORK
TITLE ==83FAN91-U1 CONTROL/ERROR RELEASE

      U     "LOG_1";
      =     L      6.0;
      U     L      6.0;
      U     #RelControlCL;
      U     #RelControlCR;
      UN    "DB_GRP_83".FAN91_PRESSURE.FM.L01_MinErr;
      U(    ;
      ON    "DB_GRP_83".FAN91_PRESSURE.FM.Alarm;
      O     "DB_GRP_83".FAN91_PRESSURE.FM.Alarm;
      )     ;
      U(    ;
      ON    "FDB_DIGIT".PRES_83FAN91_ERROR;
      O     "FDB_DIGIT".PRES_83FAN91_ERROR;
      )     ;
      UN    "DB_PROG".PRIMER.SM.CLEANING_MODE_IS_ON;
      =     #RelControl;
      U     L      6.0;
      U     #RelErrorCL;
      U     #RelErrorCR;
      =     #RelError;
NETWORK
TITLE ==83FAN91-U1 STOP DELAY AFTER 83VA51 WAS OPENED

      U     "PR_STOP_PROD_FANS";
      U     "DB_GRP_83".VA51.SM.Open;
      L     S5T#0MS;
      SE    "T_83VA51_OPENED_DELAY";
      NOP   0;
      NOP   0;
      NOP   0;
      NOP   0;
NETWORK
TITLE ==83FAN91-U1 CONTROL SIGNALS
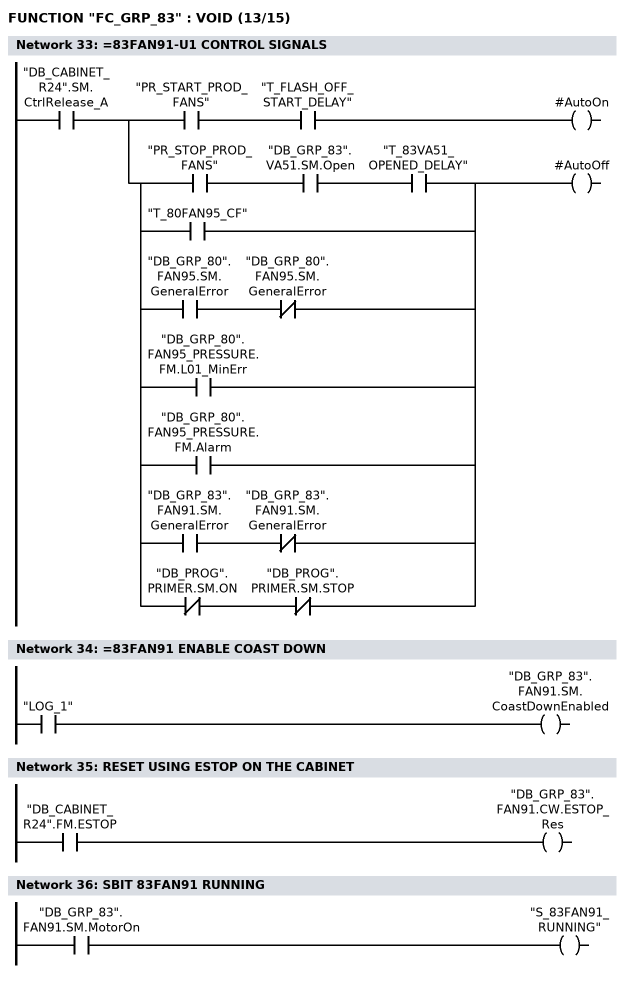
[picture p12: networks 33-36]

      U     "DB_CABINET_R24".SM.CtrlRelease_A;
      =     L      6.0;
      U     L      6.0;
      U     "PR_START_PROD_FANS";
      U     "T_FLASH_OFF_START_DELAY";
      =     #AutoOn;
      U     L      6.0;
      U(    ;
      U     "PR_STOP_PROD_FANS";
      U     "DB_GRP_83".VA51.SM.Open;
      U     "T_83VA51_OPENED_DELAY";
      O     "T_80FAN95_CF";
      O     ;
      U     "DB_GRP_80".FAN95.SM.GeneralError;
      UN    "DB_GRP_80".FAN95.SM.GeneralError;
      O     "DB_GRP_80".FAN95_PRESSURE.FM.L01_MinErr;
      O     "DB_GRP_80".FAN95_PRESSURE.FM.Alarm;
      O     ;
      U     "DB_GRP_83".FAN91.SM.GeneralError;
      UN    "DB_GRP_83".FAN91.SM.GeneralError;
      O     ;
      UN    "DB_PROG".PRIMER.SM.ON;
      UN    "DB_PROG".PRIMER.SM.STOP;
      )     ;
      =     #AutoOff;
NETWORK
TITLE ==83FAN91 ENABLE COAST DOWN

      U     "LOG_1";
      =     "DB_GRP_83".FAN91.SM.CoastDownEnabled;
NETWORK
TITLE =RESET USING ESTOP ON THE CABINET

      U     "DB_CABINET_R24".FM.ESTOP;
      =     "DB_GRP_83".FAN91.CW.ESTOP_Res;
NETWORK
TITLE =SBIT 83FAN91 RUNNING

      U     "DB_GRP_83".FAN91.SM.MotorOn;
      =     "S_83FAN91_RUNNING";
NETWORK
TITLE ==83FAN91-U1 EXHAUST AIR FAN
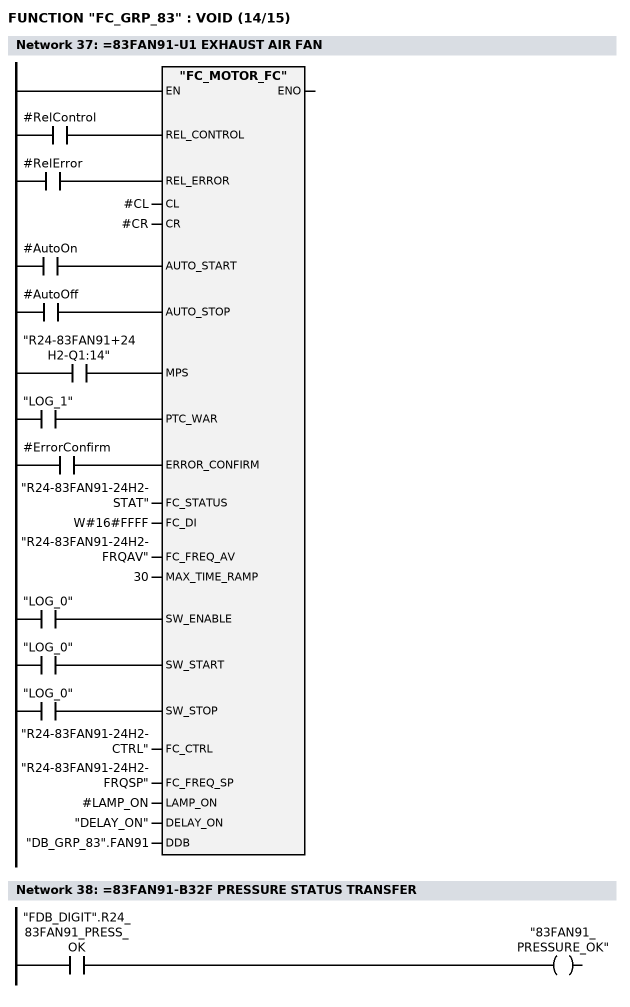
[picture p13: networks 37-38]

      U     #RelControl;
      =     L      6.0;
      BLD   103;
      U     #RelError;
      =     L      6.1;
      BLD   103;
      U     #AutoOn;
      =     L      6.2;
      BLD   103;
      U     #AutoOff;
      =     L      6.3;
      BLD   103;
      U     "R24-83FAN91+24H2-Q1:14";
      =     L      6.4;
      BLD   103;
      U     "LOG_1";
      =     L      6.5;
      BLD   103;
      U     #ErrorConfirm;
      =     L      6.6;
      BLD   103;
      U     "LOG_0";
      =     L      6.7;
      BLD   103;
      U     "LOG_0";
      =     L      7.0;
      BLD   103;
      U     "LOG_0";
      =     L      7.1;
      BLD   103;
      CALL "FC_MOTOR_FC" (
           REL_CONTROL              := L      6.0,
           REL_ERROR                := L      6.1,
           CL                       := #CL,
           CR                       := #CR,
           AUTO_START               := L      6.2,
           AUTO_STOP                := L      6.3,
           MPS                      := L      6.4,
           PTC_WAR                  := L      6.5,
           ERROR_CONFIRM            := L      6.6,
           FC_STATUS                := "R24-83FAN91-24H2-STAT",
           FC_DI                    := W#16#FFFF,
           FC_FREQ_AV               := "R24-83FAN91-24H2-FRQAV",
           MAX_TIME_RAMP            := 30,
           SW_ENABLE                := L      6.7,
           SW_START                 := L      7.0,
           SW_STOP                  := L      7.1,
           FC_CTRL                  := "R24-83FAN91-24H2-CTRL",
           FC_FREQ_SP               := "R24-83FAN91-24H2-FRQSP",
           LAMP_ON                  := #LAMP_ON,
           DELAY_ON                 := "DELAY_ON",
           DDB                      := "DB_GRP_83".FAN91);
      NOP   0;
NETWORK
TITLE ==83FAN91-B32F PRESSURE STATUS TRANSFER

      U     "FDB_DIGIT".R24_83FAN91_PRESS_OK;
      =     "83FAN91_PRESSURE_OK";
NETWORK
TITLE ==83FAN91-B32F PRESSURE MONITORING
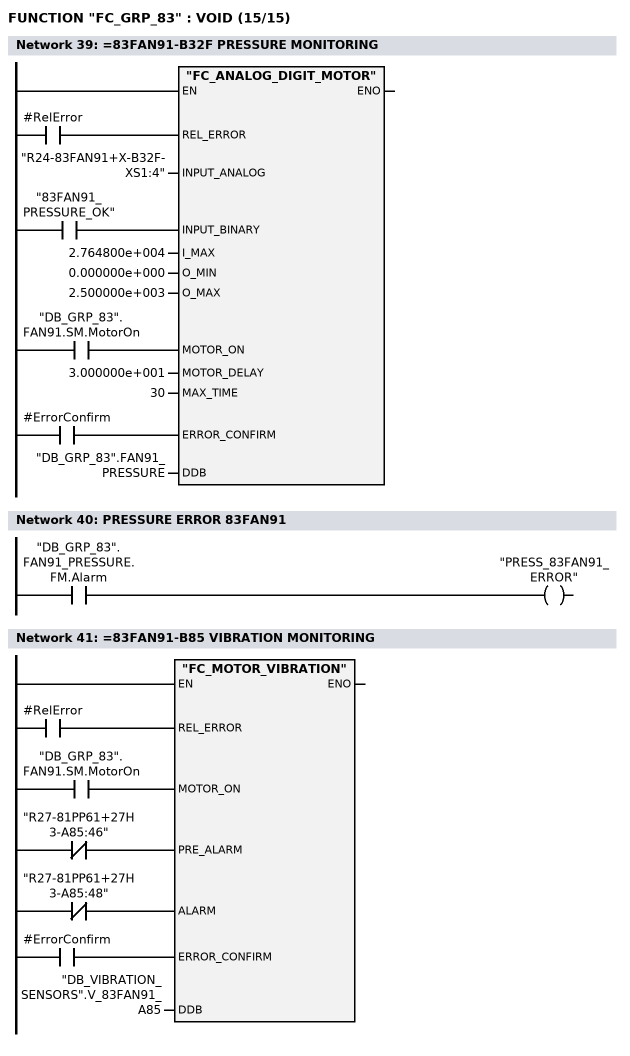
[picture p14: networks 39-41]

      U     #RelError;
      =     L      6.0;
      BLD   103;
      U     "83FAN91_PRESSURE_OK";
      =     L      6.1;
      BLD   103;
      U     "DB_GRP_83".FAN91.SM.MotorOn;
      =     L      6.2;
      BLD   103;
      U     #ErrorConfirm;
      =     L      6.3;
      BLD   103;
      CALL "FC_ANALOG_DIGIT_MOTOR" (
           REL_ERROR                := L      6.0,
           INPUT_ANALOG             := "R24-83FAN91+X-B32F-XS1:4",
           INPUT_BINARY             := L      6.1,
           I_MAX                    := 2.764800e+004,
           O_MIN                    := 0.000000e+000,
           O_MAX                    := 2.500000e+003,
           MOTOR_ON                 := L      6.2,
           MOTOR_DELAY              := 3.000000e+001,
           MAX_TIME                 := 30,
           ERROR_CONFIRM            := L      6.3,
           DDB                      := "DB_GRP_83".FAN91_PRESSURE);
      NOP   0;
NETWORK
TITLE =PRESSURE ERROR 83FAN91

      U     "DB_GRP_83".FAN91_PRESSURE.FM.Alarm;
      =     "PRESS_83FAN91_ERROR";
NETWORK
TITLE ==83FAN91-B85 VIBRATION MONITORING

      U     #RelError;
      =     L      6.0;
      BLD   103;
      U     "DB_GRP_83".FAN91.SM.MotorOn;
      =     L      6.1;
      BLD   103;
      UN    "R27-81PP61+27H3-A85:46";
      =     L      6.2;
      BLD   103;
      UN    "R27-81PP61+27H3-A85:48";
      =     L      6.3;
      BLD   103;
      U     #ErrorConfirm;
      =     L      6.4;
      BLD   103;
      CALL "FC_MOTOR_VIBRATION" (
           REL_ERROR                := L      6.0,
           MOTOR_ON                 := L      6.1,
           PRE_ALARM                := L      6.2,
           ALARM                    := L      6.3,
           ERROR_CONFIRM            := L      6.4,
           DDB                      := "DB_VIBRATION_SENSORS".V_83FAN91_A85);
      NOP   0;
NETWORK
TITLE =END



END_FUNCTION

